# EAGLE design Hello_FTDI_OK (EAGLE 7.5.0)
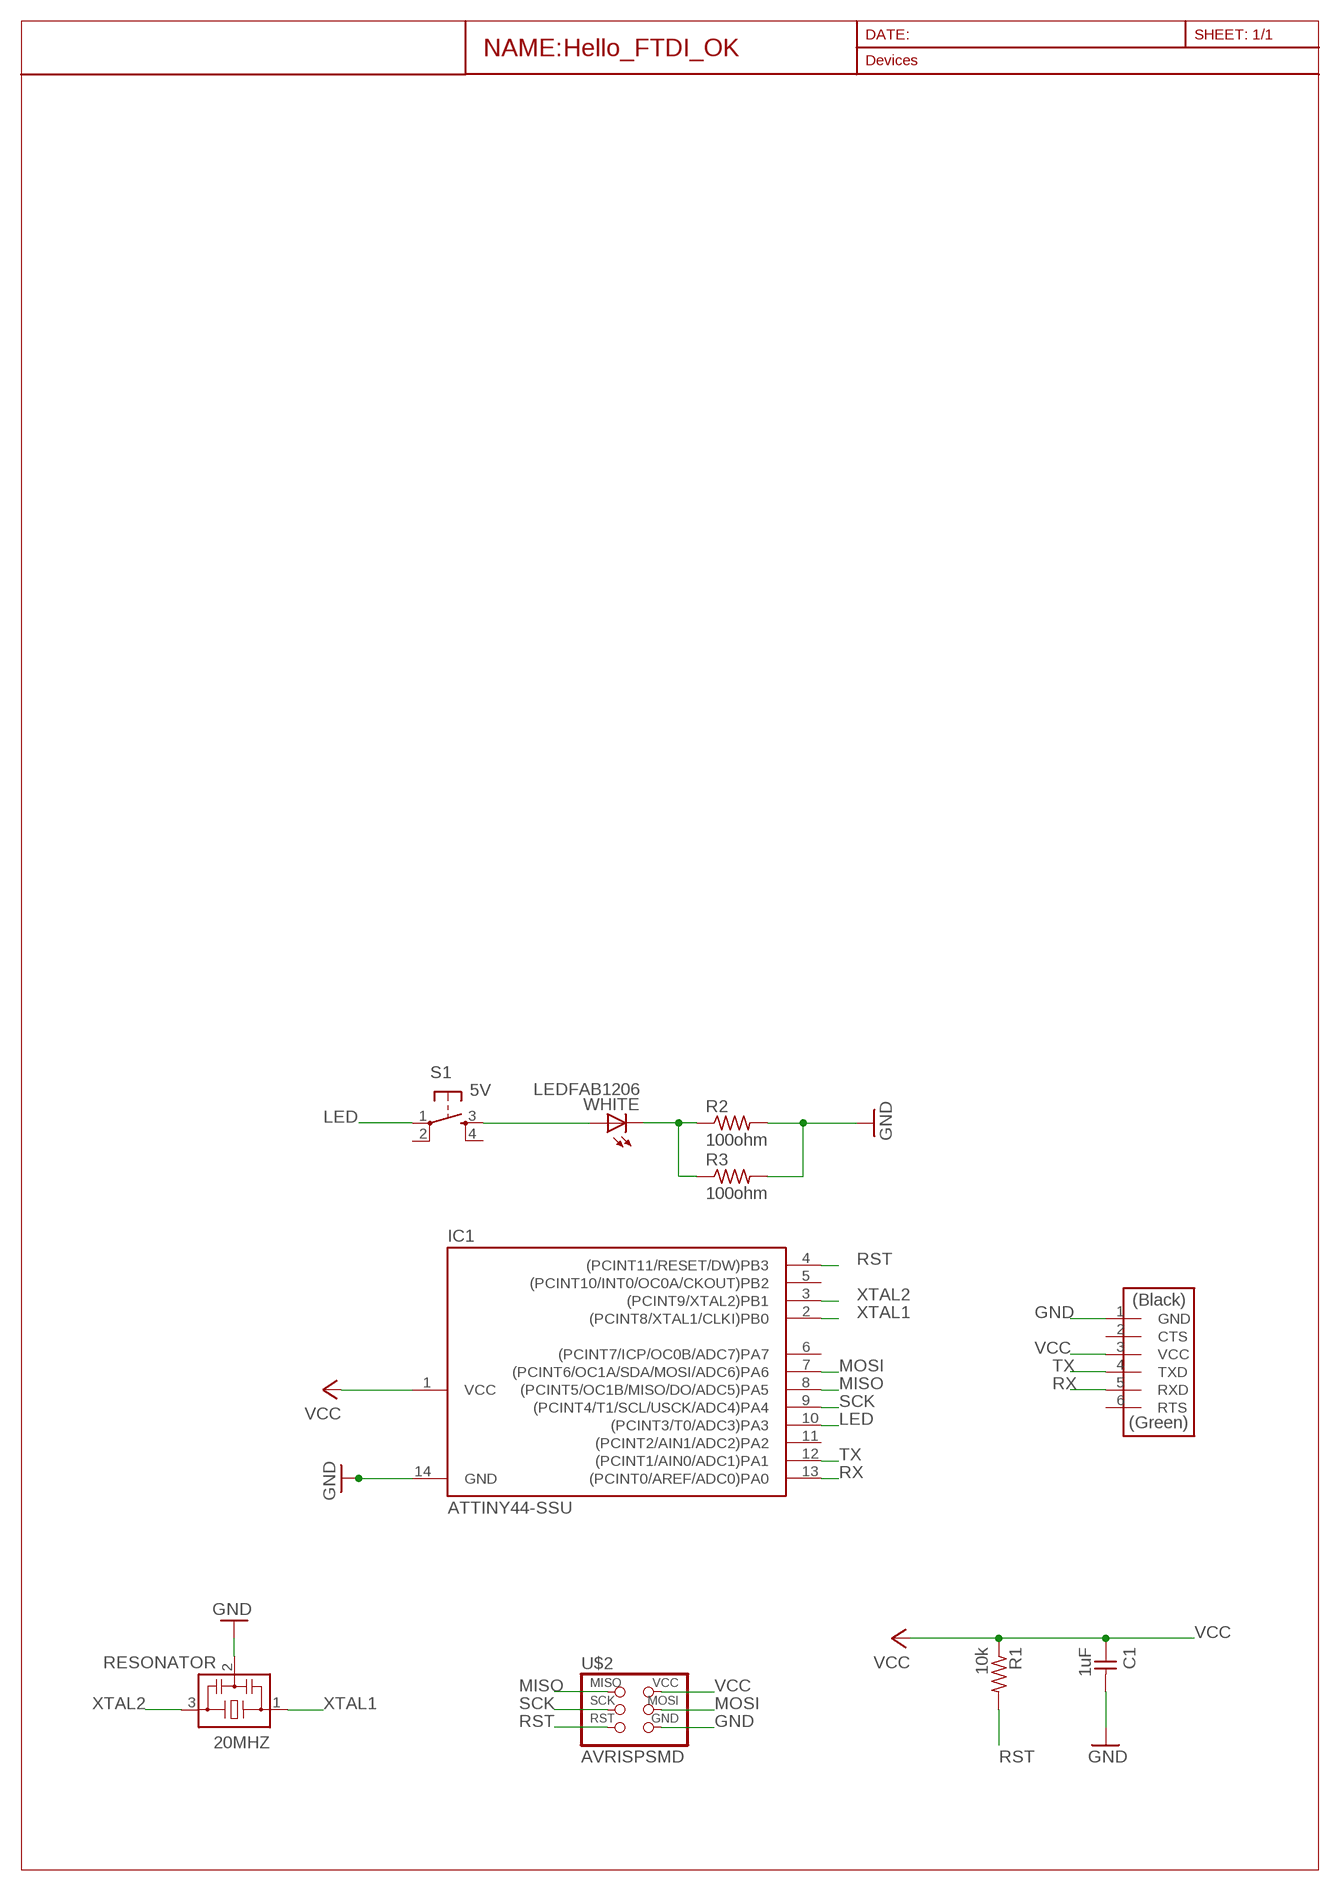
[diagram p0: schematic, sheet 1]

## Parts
20MHZ  RESONATOR  [EFOBM]
C1  1uF  CAP-UNPOLARIZEDFAB  [C1206FAB]
FTDI  FTDI-SMD-HEADER  [1X06SMD]
IC1  ATTINY44-SSU  [SOIC14]
R1  10k  RES-US1206FAB  [R1206FAB]
R2  100ohm  RES-US1206FAB  [R1206FAB]
R3  100ohm  RES-US1206FAB  [R1206FAB]
S1  5V  6MM_SWITCH6MM_SWITCH  [6MM_SWITCH]
U$2  AVRISPSMD  [2X03SMD]
WHITE  LEDFAB1206  [LED1206FAB]

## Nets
GND: 20MHZ.2 C1.2 FTDI.1(GND) IC1.14(GND) R2.2 R3.2 U$2.6(GND)
LED: IC1.10((PCINT3/T0/ADC3)PA3) S1.1(P)
MISO: IC1.8((PCINT5/OC1B/MISO/DO/ADC5)PA5) U$2.1(MISO)
MOSI: IC1.7((PCINT6/OC1A/SDA/MOSI/ADC6)PA6) U$2.4(MOSI)
N$1: R2.1 R3.1 WHITE.2(C)
N$2: S1.3(S) WHITE.1(A)
RST: IC1.4((PCINT11/RESET/DW)PB3) R1.2 U$2.5(RST)
RX: FTDI.5(RXD) IC1.13((PCINT0/AREF/ADC0)PA0)
SCK: IC1.9((PCINT4/T1/SCL/USCK/ADC4)PA4) U$2.3(SCK)
TX: FTDI.4(TXD) IC1.12((PCINT1/AIN0/ADC1)PA1)
VCC: C1.1 FTDI.3(VCC) IC1.1(VCC) R1.1 U$2.2(VCC)
XTAL1: 20MHZ.1 IC1.2((PCINT8/XTAL1/CLKI)PB0)
XTAL2: 20MHZ.3 IC1.3((PCINT9/XTAL2)PB1)
Unconnected: FTDI.2(CTS) FTDI.6(RTS) IC1.5((PCINT10/INT0/OC0A/CKOUT)PB2) IC1.6((PCINT7/ICP/OC0B/ADC7)PA7) IC1.11((PCINT2/AIN1/ADC2)PA2) S1.2(P1) S1.4(S1)

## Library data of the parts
20MHZ = fab:RESONATOR
C1 = fab:CAP-UNPOLARIZED
FTDI = fab:FTDI-SMD-HEADER
IC1 = fab:ATTINY44
R1-R3 = fab:RES-US: Resistor (US Symbol)
S1 = fab:6MM_SWITCH: OMRON SWITCH
U$2 = fab:AVRISP
WHITE = fab:LED: LED

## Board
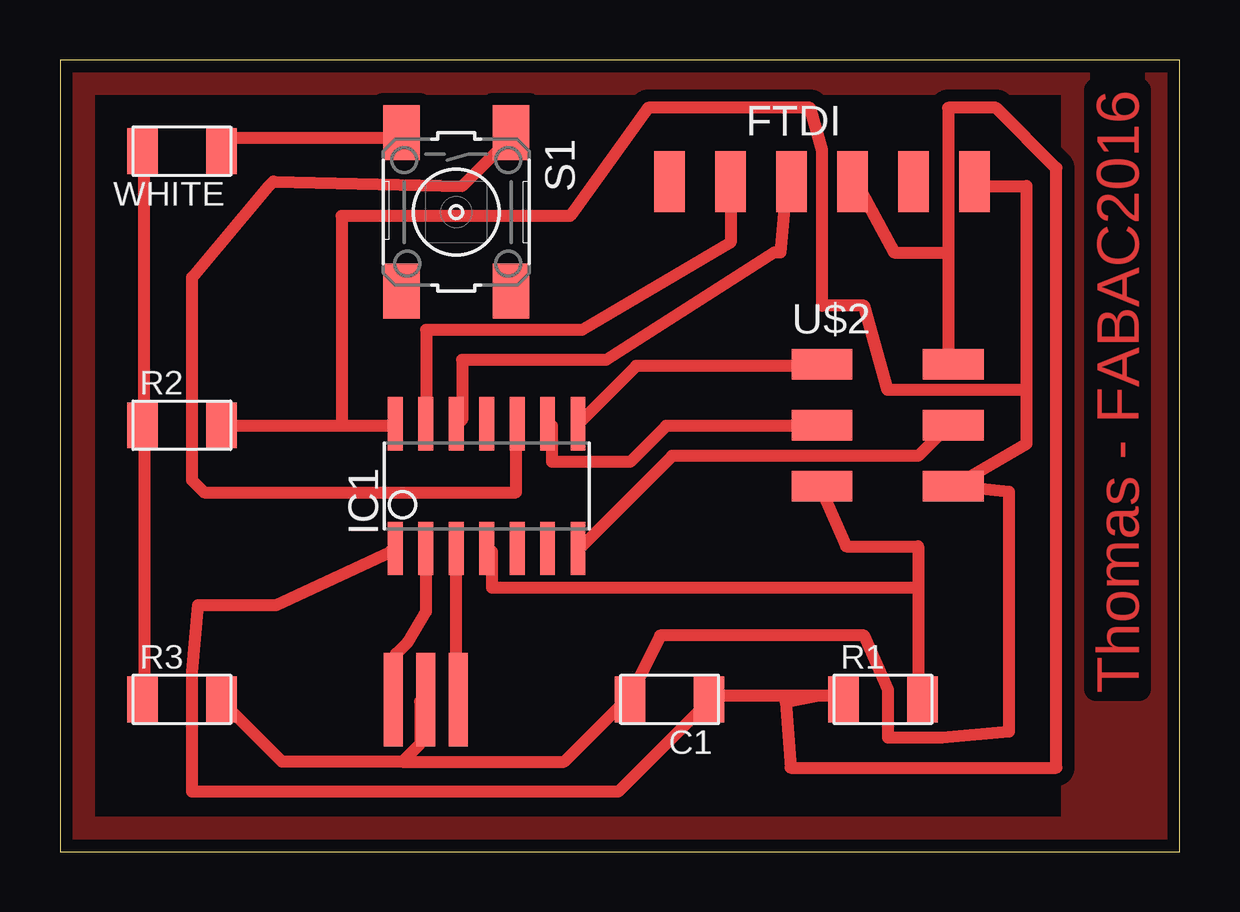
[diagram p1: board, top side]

Size 46.66 x 33.01 mm. Coordinates in mm from the lower left corner, seen from the top.
Outline: 0,0 46.66,0 46.66,33.01 0,33.01 0,0
Copper layers (1*16): Top 0.035mm / dielectric 1.5mm / Bottom 0.035mm
Design rules "SeeedStudio_2layer_DRU_no_angle_20140221 *": minimum track width 20mil, minimum drill 12mil, track to track 20mil, track to pad 6mil, pad to pad 6mil, via to via 6mil, smd to smd 0mil, copper to edge 20mil, drill to drill 10mil, minimum pad ring 10mil, minimum via ring 6mil, stop-mask expansion 2mil, vias tented up to drill 100mil, thermal gap 10mil

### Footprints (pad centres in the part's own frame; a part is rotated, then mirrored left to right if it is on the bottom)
EFOBM = smd 0.8 x 3.9: 1 -1.35,0; 2 0,0; 3 1.35,0
C1206FAB = smd 1.27 x 1.905: 1 -1.651,0; 2 1.651,0
1X06SMD = smd 2.54 x 1.27: 1 0,6.35; 2 0,3.81; 3 0,1.27; 4 0,-1.27; 5 0,-3.81; 6 0,-6.35
SOIC14 = smd 0.61 x 2.21: 1 -3.81,-2.603; 2 -2.54,-2.603; 3 -1.27,-2.603; 4 0,-2.603; 5 1.27,-2.603; 6 2.54,-2.603; 7 3.81,-2.603; 8 3.81,2.603; 9 2.54,2.603; 10 1.27,2.603; 11 0,2.603; 12 -1.27,2.603; 13 -2.54,2.603; 14 -3.81,2.603
R1206FAB = smd 1.27 x 1.905: 1 -1.651,0; 2 1.651,0
6MM_SWITCH = smd 2.286 x 1.524: 1 -3.302,2.286; 2 3.302,2.286; 3 -3.302,-2.286; 4 3.302,-2.286
2X03SMD = smd 2.54 x 1.27: 1 -2.54,2.54; 2 2.92,2.54; 3 -2.54,0; 4 2.92,0; 5 -2.54,-2.54; 6 2.92,-2.54
LED1206FAB = smd 1.27 x 1.905: 1 -1.651,0; 2 1.651,0

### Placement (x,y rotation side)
20MHZ  15.24,6.35 0 top
C1  25.4,6.35 180 top
FTDI  31.75,27.94 270 top
IC1  17.78,15.24 0 top
R1  34.29,6.35 0 top
R2  5.08,17.78 0 top
R3  5.08,6.35 0 top
S1  16.51,26.67 270 top
U$2  34.29,17.78 0 top
WHITE  5.08,29.21 180 top

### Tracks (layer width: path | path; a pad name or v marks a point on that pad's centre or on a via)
GND
  Top 0.508: 14.25,3.75 9.25,3.75 6.75,6.25 R3.2 | 14.25,3.75 15,4.5 15,6.25 20MHZ.2 | 14.25,3.75 21,3.75 23.5,6.25 C1.2 23.75,6.5 25,9.02 33.5,9.02 34.5,6.75 34.5,4.75 36.75,4.75 39.54,5 39.54,15 U$2.6 37.25,15.25 40.27,17 40.27,19.25 | 11.73,17.75 13.75,17.75 IC1.14 | 11.73,17.75 6.75,17.75 R2.2 | 40.27,19.25 40.27,27.75 38.25,27.75 FTDI.1 | 11.73,17.75 11.73,26.5 21.25,26.5 24.5,31.02 31.25,31.02 31.75,29.25 31.75,22.77 33.5,22.77 34.48,19.25 40.27,19.25
LED
  Top 0.508: IC1.10 19,17.75 19,14.98 6,14.98 5.5,15.48 5.5,23.94 8.7,27.75 8.89,27.94 16.75,27.75 18.75,29.75 S1.1
MISO
  Top 0.508: IC1.8 21.75,18 24,20.25 31.75,20.25 U$2.1
MOSI
  Top 0.508: IC1.7 21.75,12.75 25.5,16.5 35.75,16.5 37,17.75 U$2.4
N$1
  Top 0.508: R3.1 3.5,6.5 3.5,17.75 R2.1 3.5,18 3.5,29 WHITE.2
N$2
  Top 0.508: WHITE.1 6.75,29.25 7.25,29.75 14,29.75 S1.3
N$3
  pour Top: 0,1.27 46.99,1.27 46.99,0 0,0
N$4
  pour Top: 1.27,33.02 0,33.02 0,0 1.27,0
N$5
  pour Top: 41.91,33.02 41.91,0 46.99,0 46.99,33.02
N$6
  pour Top: 0,33.02 41.91,33.02 41.91,31.75 0,31.75
RST
  Top 0.508: 35.75,11 35.75,12.73 32.75,12.73 31.75,15 U$2.5 | 35.75,11 35.75,6.5 R1.2 | 35.75,11 18,11 18,12.5 IC1.4
RX
  Top 0.508: FTDI.5 27.94,25.4 21.75,21.75 15.25,21.75 15.25,18 IC1.13
SCK
  Top 0.508: IC1.9 20.5,17.75 20.5,16.25 23.75,16.25 25.25,17.75 31.75,17.75 U$2.3
TX
  Top 0.508: IC1.12 16.75,18 16.75,20.5 22.75,20.5 29.77,24.98 30.02,24.98 30.25,27.75 FTDI.4
VCC
  Top 0.508: 37,24.98 37,20.5 U$2.2 | 37,24.98 34.75,24.98 33.25,27.75 FTDI.3 | 31.5,6.5 32.5,6.5 R1.1 | 31.5,6.5 27.25,6.5 C1.1 27,6.25 23.25,2.5 5.5,2.5 5.5,7.5 5.75,10.29 9,10.29 13.75,12.5 IC1.1 | 37,24.98 37,31.02 39,31.02 41.52,28.5 41.52,3.5 30.44,3.5 30.23,6.25 31.5,6.5
XTAL1
  Top 0.508: IC1.2 15.25,12.5 15.25,10.02 14.5,8.75 14,8.25 14,6.5 20MHZ.1
XTAL2
  Top 0.508: IC1.3 16.5,12.5 16.5,6.5 20MHZ.3

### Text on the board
Top: Thomas - FABAC2016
